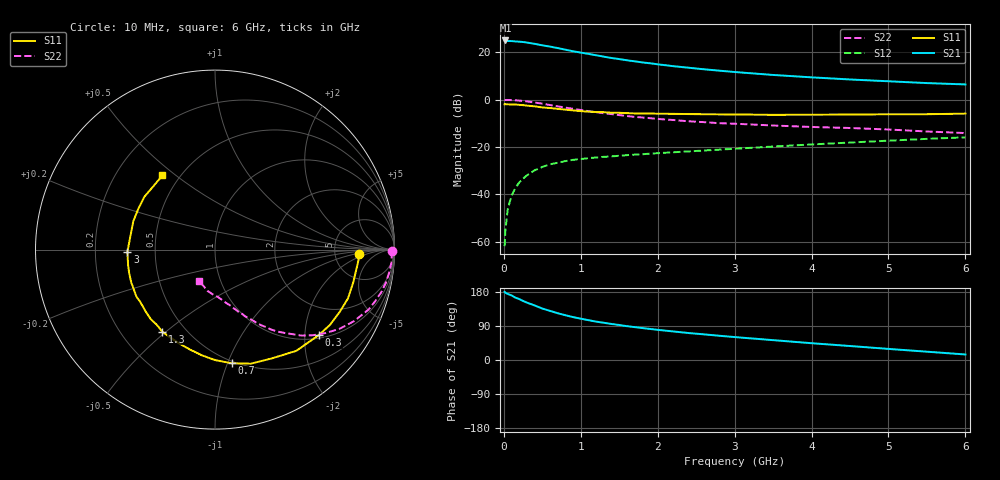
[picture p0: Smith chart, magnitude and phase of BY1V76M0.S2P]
! SIEMENS Small Signal Semiconductors
! BFY420
! Si NPN RF SIEGET Grounded Emitter Transistor in MICRO-X
! VCE = 1.75 V  IC = 6 mA
! Common Emitter S-Parameters:  October  1996
# GHz  S  MA  R  50
!  f  S11  S21  S12  S22
! GHz  MAG  ANG  MAG  ANG  MAG  ANG  MAG  ANG
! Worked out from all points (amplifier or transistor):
!   36 points, 10 MHz to 6 GHz, reference 50 ohm
!   highest |S21| = 25.0 dB at 20 MHz (marker M1)
!   |S21| within 3 dB of that: start of sweep to 665.2 MHz
!   unconditionally stable (mu >= 1): 2.976 GHz to end of sweep
!   at 250 MHz: K = 0.12, MSG = 28.9 dB, |S12| = -33.4 dB
!   at 1.4 GHz: K = 0.60, MSG = 20.8 dB, |S12| = -24.0 dB
!   at 6 GHz: K = 1.14, MAG = 8.9 dB, |S12| = -15.9 dB
!   S11 on the Smith chart (normalised r, x): 10 MHz: 8.86, -1.10; 300 MHz: 1.09, -2.36; 700 MHz: 0.48, -1.03; 1.3 GHz: 0.37, -0.48; 3 GHz: 0.34, -0.01; 6 GHz: 0.40, +0.45
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0.01  0.8 -1.6  17.84 179.8  0.0008 105.5  0.9889 -0.6
0.02  0.8039 -3.0  17.85 177.4  0.0017 89.0  0.9842 -1.4
0.05  0.7971 -6.6  17.38 174.4  0.0048 84.9  0.987 -3.7
0.1  0.7916 -13.5  17.33 170.4  0.0093 86.1  0.9792 -7.4
0.15  0.7893 -20.1  17.03 164.6  0.0135 78.0  0.9692 -11.1
0.2  0.7767 -26.6  16.83 160.8  0.0178 76.7  0.9562 -14.4
0.25  0.7658 -33.2  16.55 155.9  0.0214 73.3  0.9369 -18.0
0.3  0.7493 -39.4  16.11 151.4  0.0252 69.9  0.9186 -21.3
0.4  0.7235 -51.2  15.17 144.0  0.0321 65.0  0.8714 -27.2
0.5  0.6842 -62.3  14.1 135.8  0.0379 60.3  0.822 -32.5
0.6  0.666 -72.6  13.23 129.6  0.043 56.2  0.771 -37.1
0.7  0.64 -81.7  12.34 123.5  0.0464 52.8  0.7245 -41.2
0.9  0.593 -97.3  10.56 113.2  0.0535 47.3  0.6402 -47.4
1.1  0.5588 -111.4  9.282 105.1  0.0581 44.5  0.5727 -52.8
1.3  0.5434 -122.8  8.117 98.2  0.0619 42.1  0.5162 -56.7
1.7  0.5126 -141.3  6.469 86.8  0.0689 39.8  0.433 -63.0
2.2  0.5013 -158.4  5.11 75.4  0.0773 37.9  0.3718 -69.2
3  0.4879 -178.7  3.843 60.5  0.0917 36.2  0.3102 -77.1
3.5  0.4772 170.7  3.33 52.4  0.1021 34.7  0.2847 -81.7
4.5  0.484 152.0  2.673 36.9  0.1241 30.1  0.252 -92.1
5.5  0.4929 133.7  2.242 21.9  0.1484 23.8  0.2126 -107.5
6  0.507 125.4  2.101 14.6  0.1601 20.2  0.1968 -117.7
